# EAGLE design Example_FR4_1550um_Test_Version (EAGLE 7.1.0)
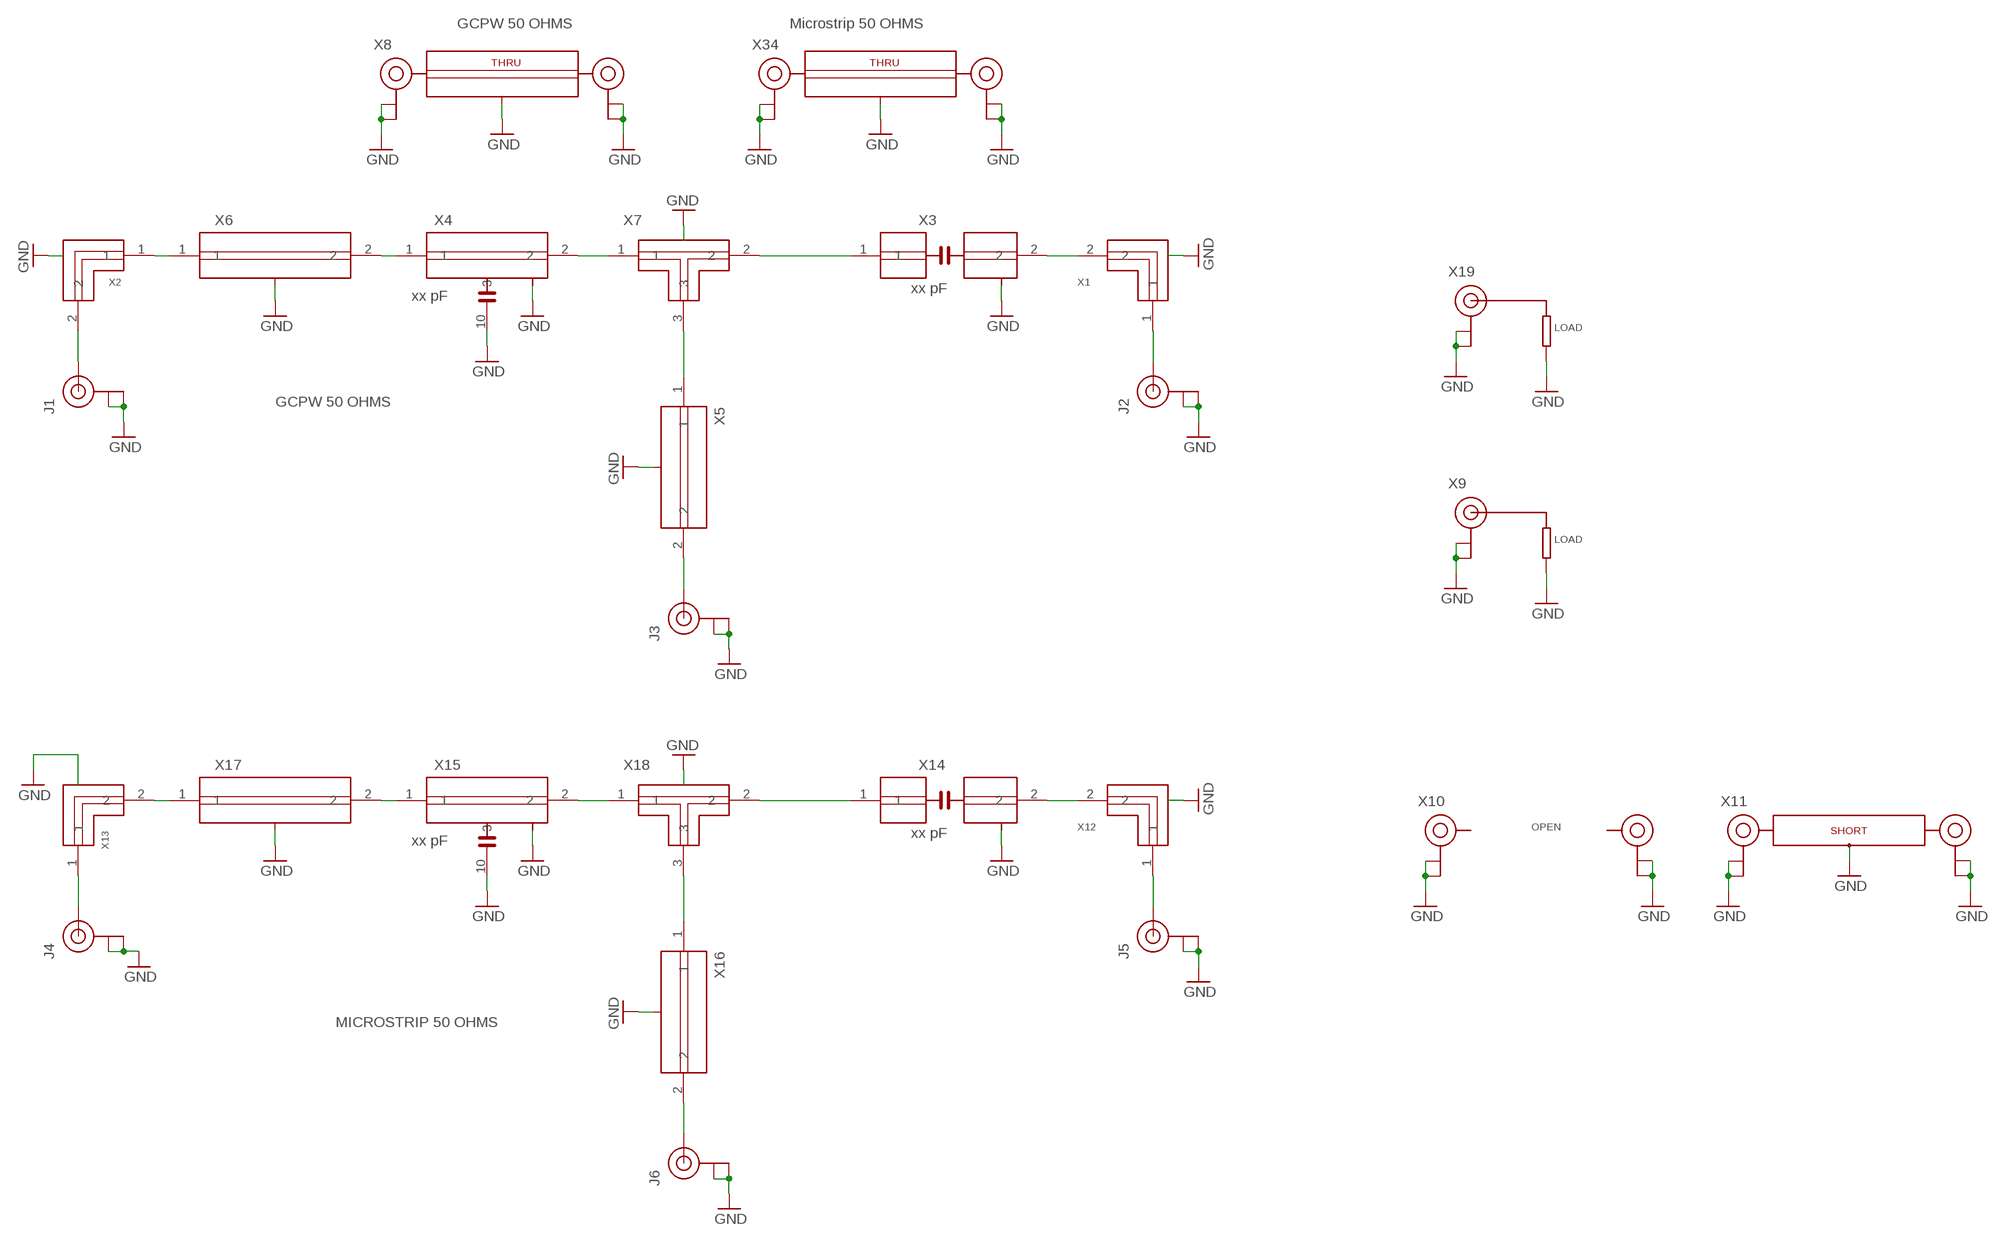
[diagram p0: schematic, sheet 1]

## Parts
J1  U.FL  [U.FL]
J2  U.FL  [U.FL]
J3  U.FL  [U.FL]
J4  U.FL  [U.FL]
J5  U.FL  [U.FL]
J6  U.FL  [U.FL]
X1  CHIPDESIGN_GCPW_50_OHM_L  [GCPW_50_OHM_LEFT]
X2  CHIPDESIGN_GCPW_50_OHM_R  [GCPW_50_OHM_RIGHT]
X3  xx pF  CHIPDESIGN_GCPW_50_OHM_SERIES_0402  [GCPW_50_OHM_0402_SERIES]
X4  xx pF  CHIPDESIGN_GCPW_50_OHM_SHUNT_0402  [GCPW_50_OHM_0402_SHUNT]
X5  CHIPDESIGN_GCPW_50_OHM_TLINE_SHORT  [GCPW_50_OHM_TLINE_SHORT]
X6  CHIPDESIGN_GCPW_50_OHM_TLINE_LONG  [GCPW_50_OHM_TLINE_LONG]
X7  CHIPDESIGN_GCPW_50_OHM_TJUNCTION  [GCPW_50_OHM_TEE]
X8  CHIPDESIGN_GCPW_50_OHM_THRU  [GCPW_50_OHM_THRU]
X9  LOAD_GCPW  [LOAD_GCPW]
X10  OPEN  [OPEN]
X11  SHORT  [SHORT]
X12  CHIPDESIGN_MICROSTRIP_50_OHM_L  [MICROSTRIP_50_OHM_LEFT]
X13  CHIPDESIGN_MICROSTRIP_50_OHM_R  [MICROSTRIP_50_OHM_RIGHT]
X14  xx pF  CHIPDESIGN_MICROSTRIP_50_OHM_SERIES_0402  [MICROSTRIP_50_OHM_0402_SERIES]
X15  xx pF  CHIPDESIGN_MICROSTRIP_50_OHM_SHUNT_0402  [MICROSTRIP_50_OHM_0402_SHUNT]
X16  CHIPDESIGN_MICROSTRIP_50_OHM_TLINE_SHORT  [MICROSTRIP_50_OHM_TLINE_SHORT]
X17  CHIPDESIGN_MICROSTRIP_50_OHM_TLINE_LONG  [MICROSTRIP_50_OHM_TLINE_LONG]
X18  CHIPDESIGN_MICROSTRIP_50_OHM_TJUNCTION  [MICROSTRIP_50_OHM_TEE]
X19  LOAD_MICROSTRIP  [LOAD_MICROSTRIP]
X34  CHIPDESIGN_MICROSTRIP_50_OHM_THRU  [MICROSTRIP_50_OHM_THRU]

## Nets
GND: J1.P$1(GND) J1.P$2(GND) J2.P$1(GND) J2.P$2(GND) J3.P$1(GND) J3.P$2(GND) J4.P$1(GND) J4.P$2(GND) J5.P$1(GND) J5.P$2(GND) J6.P$1(GND) J6.P$2(GND) X1.3(GND) X1.4(GND) X1.5(GND) X1.6(GND) X1.7(GND) X1.8(GND) X1.9(GND) X1.10(GND) X2.3(GND) X2.4(GND) X2.5(GND) X2.6(GND) X2.7(GND) X2.8(GND) X2.9(GND) X2.10(GND) X3.3(GND) X3.4(GND) X3.5(GND) X3.6(GND) X3.7(GND) X3.8(GND) X3.9(GND) X3.10(GND) X3.11(GND) X3.12(GND) X4.3(GND) X4.4(GND) X4.5(GND) X4.6(GND) X4.7(GND) X4.8(GND) X4.9(GND) X4.10 X4.11(GND) X4.12(GND) X5.3(GND) X5.4(GND) X5.5(GND) X5.6(GND) X6.3(GND) X6.4(GND) X6.5(GND) X6.6(GND) X6.7(GND) X6.8(GND) X6.9(GND) X6.10(GND) X6.11(GND) X6.12(GND) X7.4(GND) X7.5(GND) X7.6(GND) X7.7(GND) X7.8(GND) X7.9(GND) X7.10(GND) X7.11(GND) X7.12(GND) X7.13(GND) X7.14(GND) X8.3(GND) X8.4(GND) X8.5(GND) X8.6(GND) X8.7(GND) X8.8(GND) X8.9(GND) X8.10(GND) X8.11(GND) X8.12(GND) X8.P$1(GND) X8.P$2(GND) X8.P$5(GND) X8.P$6(GND) X9.P$1(GND) X9.P$2(GND) X9.P$6(GND) X9.P$7(GND) X9.P$8(GND) X9.P$9(GND) X9.P$10(GND) X9.P$11(GND) X9.P$12(GND) X10.1(GND) X10.2(GND) X10.3(GND) X10.4(GND) X10.5(GND) X10.6(GND) X10.7(GND) X10.8(GND) X10.9(GND) X10.10(GND) X10.11(GND) X10.12(GND) X10.13(GND) X10.14(GND) X10.15(GND) X10.16(GND) X10.17(GND) X10.18(GND) X10.19(GND) X10.20(GND) X10.21(GND) X10.22(GND) X10.23(GND) X10.24(GND) X11.P$1(GND) X11.P$2(GND) X11.P$3(GND) X11.P$5(GND) X11.P$6(GND) X11.P$7(GND) X12.P$1(GND) X12.P$2(GND) X12.P$3(GND) X12.P$4(GND) X12.P$5(GND) X12.P$6(GND) X12.P$7(GND) X12.P$8(GND) X12.P$9(GND) X13.P$1(GND) X13.P$2(GND) X13.P$3(GND) X13.P$4(GND) X13.P$5(GND) X13.P$7(GND) X13.P$8(GND) X13.P$15(GND) X13.P$16(GND) X14.P$1(GND) X14.P$2(GND) X14.P$3(GND) X14.P$4(GND) X14.P$5(GND) X14.P$6(GND) X14.P$7(GND) X14.P$8(GND) X14.P$9(GND) X14.P$10(GND) X15.10 X15.P$1(GND) X15.P$2(GND) X15.P$3(GND) X15.P$4(GND) X15.P$5(GND) X15.P$6(GND) X15.P$7(GND) X15.P$8(GND) X15.P$9(GND) X16.P$1(GND) X16.P$2(GND) X16.P$3(GND) X16.P$4(GND) X17.P$1(GND) X17.P$2(GND) X17.P$3(GND) X17.P$4(GND) X17.P$5(GND) X17.P$6(GND) X17.P$7(GND) X17.P$8(GND) X17.P$9(GND) X17.P$10(GND) X18.P$1(GND) X18.P$2(GND) X18.P$3(GND) X18.P$4(GND) X18.P$5(GND) X18.P$6(GND) X18.P$7(GND) X19.P$1(GND) X19.P$2(GND) X19.P$6(GND) X19.P$7(GND) X19.P$8(GND) X19.P$9(GND) X19.P$10(GND) X19.P$11(GND) X19.P$12(GND) X34.1(GND) X34.2(GND) X34.3(GND) X34.4(GND) X34.5(GND) X34.6(GND) X34.7(GND) X34.8(GND) X34.9(GND) X34.10(GND) X34.11(GND) X34.12(GND) X34.13(GND) X34.14(GND) X34.15(GND) X34.16(GND) X34.17(GND) X34.18(GND) X34.P$1(GND) X34.P$2(GND) X34.P$5(GND) X34.P$6(GND)
N$1: J1.P$3(SIGNAL) X2.2
N$2: X2.1 X6.1
N$3: X4.1 X6.2
N$4: X4.2 X7.1
N$5: X3.1 X7.2
N$6: X5.1 X7.3
N$7: J3.P$3(SIGNAL) X5.2
N$8: X1.2 X3.2
N$9: J2.P$3(SIGNAL) X1.1
N$10: X13.2 X17.1
N$11: J4.P$3(SIGNAL) X13.1
N$13: X15.1 X17.2
N$14: X15.2 X18.1
N$15: X14.1 X18.2
N$16: X16.1 X18.3
N$17: J6.P$3(SIGNAL) X16.2
N$18: X12.2 X14.2
N$19: J5.P$3(SIGNAL) X12.1

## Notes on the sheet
- GCPW 50 OHMS | Microstrip 50 OHMS
- GCPW 50 OHMS
- MICROSTRIP 50 OHMS

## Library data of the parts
J1-J6 = Chipdesign_Isola_050:U.FL: SMD antenna connector- WRL-09144; MPN: U.FL-R-SMT-1(10); OC_NEWARK: 50P8856; PROD_ID: CONN-09193
X1 = Chipdesign_FR4_050:CHIPDESIGN_GCPW_50_OHM_L: Grounded Coplanar Waveguide Line - left; Relative dielectric constant = 4.4; Thickness of dielectric = 1.55mm.; DIELECTRIC: FR4; DK: 4.4; E_EFF: 2.78; OC_NEWARK: unknown; PCB_THICKNESS: 1.55MM; ZO: 50 ohms
X2 = Chipdesign_FR4_050:CHIPDESIGN_GCPW_50_OHM_R: Grounded Coplanar Waveguide Line - right; Relative dielectric constant = 4.4; Thickness of dielectric = 1.55mm.; DIELECTRIC: FR4; DK: 4.4; E_EFF: 2.78; OC_NEWARK: unknown; PCB_THICKNESS: 1.55MM; ZO: 50 ohms
X3 = Chipdesign_FR4_050:CHIPDESIGN_GCPW_50_OHM_SERIES_0402: Grounded Coplanar Waveguide Line - series cap 0402; Relative dielectric constant = 4.4; Thickness of dielectric = 1.55mm.; DIELECTRIC: FR4; DK: 4.4; E_EFF: 2.78; OC_NEWARK: unknown; PCB_THICKNESS: 1.55MM; ZO: 50 ohms
X4 = Chipdesign_FR4_050:CHIPDESIGN_GCPW_50_OHM_SHUNT_0402: Grounded Coplanar Waveguide Line - shunt cap 0402; Relative dielectric constant = 4.4; Thickness of dielectric = 1.55mm.; DIELECTRIC: FR4; DK: 4.4; E_EFF: 2.78; OC_NEWARK: unknown; PCB_THICKNESS: 1.55MM; ZO: 50 ohms
X5 = Chipdesign_FR4_050:CHIPDESIGN_GCPW_50_OHM_TLINE_SHORT: Grounded Coplanar Waveguide Line - TLINE; Relative dielectric constant = 4.4; Thickness of dielectric = 1.55mm.; DIELECTRIC: FR4; DK: 4.4; E_EFF: 2.78; OC_NEWARK: unknown; PCB_THICKNESS: 1.55MM; ZO: 50 Ohms
X6 = Chipdesign_FR4_050:CHIPDESIGN_GCPW_50_OHM_TLINE_LONG: Grounded Coplanar Waveguide Line - TLINE, long; Relative dielectric constant = 4.4; Thickness of dielectric = 1.55mm.; DIELECTRIC: FR4; DK: 4.4; E_EFF: 2.78; OC_NEWARK: unknown; PCB_THICKNESS: 1.55MM; ZO: 50 ohms
X7 = Chipdesign_FR4_050:CHIPDESIGN_GCPW_50_OHM_TJUNCTION: Grounded Coplanar Waveguide - T JUNCTION, long; Relative dielectric constant = 4.4; Thickness of dielectric = 1.55mm.; DIELECTRIC: FR4; DK: 4.4; E_EFF: 2.78; OC_NEWARK: unknown; PCB_THICKNESS: 1.55MM; ZO: 50 ohms
X8 = Chipdesign_FR4_050:CHIPDESIGN_GCPW_50_OHM_THRU: Relative dielectric constant = 4.4; Thickness of dielectric = 1.55mm.; DIELECTRIC: FR4; DK: 4.4; E_EFF: 2.78; OC_NEWARK: unknown; PCB_THICKNESS: 1.55MM; ZO: 50 ohms
X9 = Chipdesign_FR4_050:LOAD_GCPW: Relative dielectric constant = 4.4; Thickness of dielectric = 1.55mm.; OC_NEWARK: unknown
X10 = Chipdesign_FR4_050:OPEN; OC_NEWARK: unknown
X11 = Chipdesign_FR4_050:SHORT: Relative dielectric constant = 4.4; Thickness of dielectric = 1.55mm.; OC_NEWARK: unknown
X12 = Chipdesign_FR4_050:CHIPDESIGN_MICROSTRIP_50_OHM_L: Grounded Coplanar Waveguide Line - left; Relative dielectric constant = 4.4; Thickness of dielectric = 1.55mm.; DIELECTRIC: FR4; DK: 4.4; OC_NEWARK: unknown; PCB_THICKNESS: 1.55MM; TRACK_THICKNESS: 35um; ZO: 50 ohms
X13 = Chipdesign_FR4_050:CHIPDESIGN_MICROSTRIP_50_OHM_R: Grounded Coplanar Waveguide Line - right; Relative dielectric constant = 4.4; Thickness of dielectric = 1.55mm.; DIELECTRIC: FR4; DK: 4.4; OC_NEWARK: unknown; PCB_THICKNESS: 1.55MM; TRACK_THICKNESS: 35um; ZO: 50 ohms
X14 = Chipdesign_FR4_050:CHIPDESIGN_MICROSTRIP_50_OHM_SERIES_0402: Grounded Coplanar Waveguide Line - series cap 0402; Relative dielectric constant = 4.4; Thickness of dielectric = 1.55mm.; DIELECTRIC: FR4; DK: 4.4; OC_NEWARK: unknown; PCB_THICKNESS: 1.55MM; TRACK_THICKNESS: 35um; ZO: 50 ohms
X15 = Chipdesign_FR4_050:CHIPDESIGN_MICROSTRIP_50_OHM_SHUNT_0402: Grounded Coplanar Waveguide Line - shunt cap 0402; Relative dielectric constant = 4.4; Thickness of dielectric = 1.55mm.; DIELECTRIC: FR4; DK: 4.4; OC_NEWARK: unknown; PCB_THICKNESS: 1.55MM; TRACK_THICKNESS: 35um; ZO: 50 ohms
X16 = Chipdesign_FR4_050:CHIPDESIGN_MICROSTRIP_50_OHM_TLINE_SHORT: Grounded Coplanar Waveguide Line - TLINE; Relative dielectric constant = 4.4; Thickness of dielectric = 1.55mm.; DIELECTRIC: FR4; DK: 4.4; OC_NEWARK: unknown; PCB_THICKNESS: 1.55MM; TRACK_THICKNESS: 35um; ZO: 50 ohms
X17 = Chipdesign_FR4_050:CHIPDESIGN_MICROSTRIP_50_OHM_TLINE_LONG: Grounded Coplanar Waveguide Line - TLINE, long; Relative dielectric constant = 4.4; Thickness of dielectric = 1.55mm.; DIELECTRIC: FR4; DK: 4.4; OC_NEWARK: unknown; PCB_THICKNESS: 1.55MM; TRACK_THICKNESS: 35um; ZO: 50 ohms
X18 = Chipdesign_FR4_050:CHIPDESIGN_MICROSTRIP_50_OHM_TJUNCTION: Grounded Coplanar Waveguide - T JUNCTION, long; Relative dielectric constant = 4.4; Thickness of dielectric = 1.55mm.; DIELECTRIC: FR4; DK: 4.4; OC_NEWARK: unknown; PCB_THICKNESS: 1.55MM; TRACK_THICKNESS: 35um; ZO: 50 ohms
X19 = Chipdesign_FR4_050:LOAD_MICROSTRIP: Relative dielectric constant = 4.4; Thickness of dielectric = 1.55mm.; OC_NEWARK: unknown
X34 = Chipdesign_FR4_050:CHIPDESIGN_MICROSTRIP_50_OHM_THRU: Relative dielectric constant = 4.4; Thickness of dielectric = 1.55mm.; DIELECTRIC: FR4; DK: 4.4; OC_NEWARK: unknown; PCB_THICKNESS: 1.55MM; TRACK_THICKNESS: 35um; ZO: 50 ohms

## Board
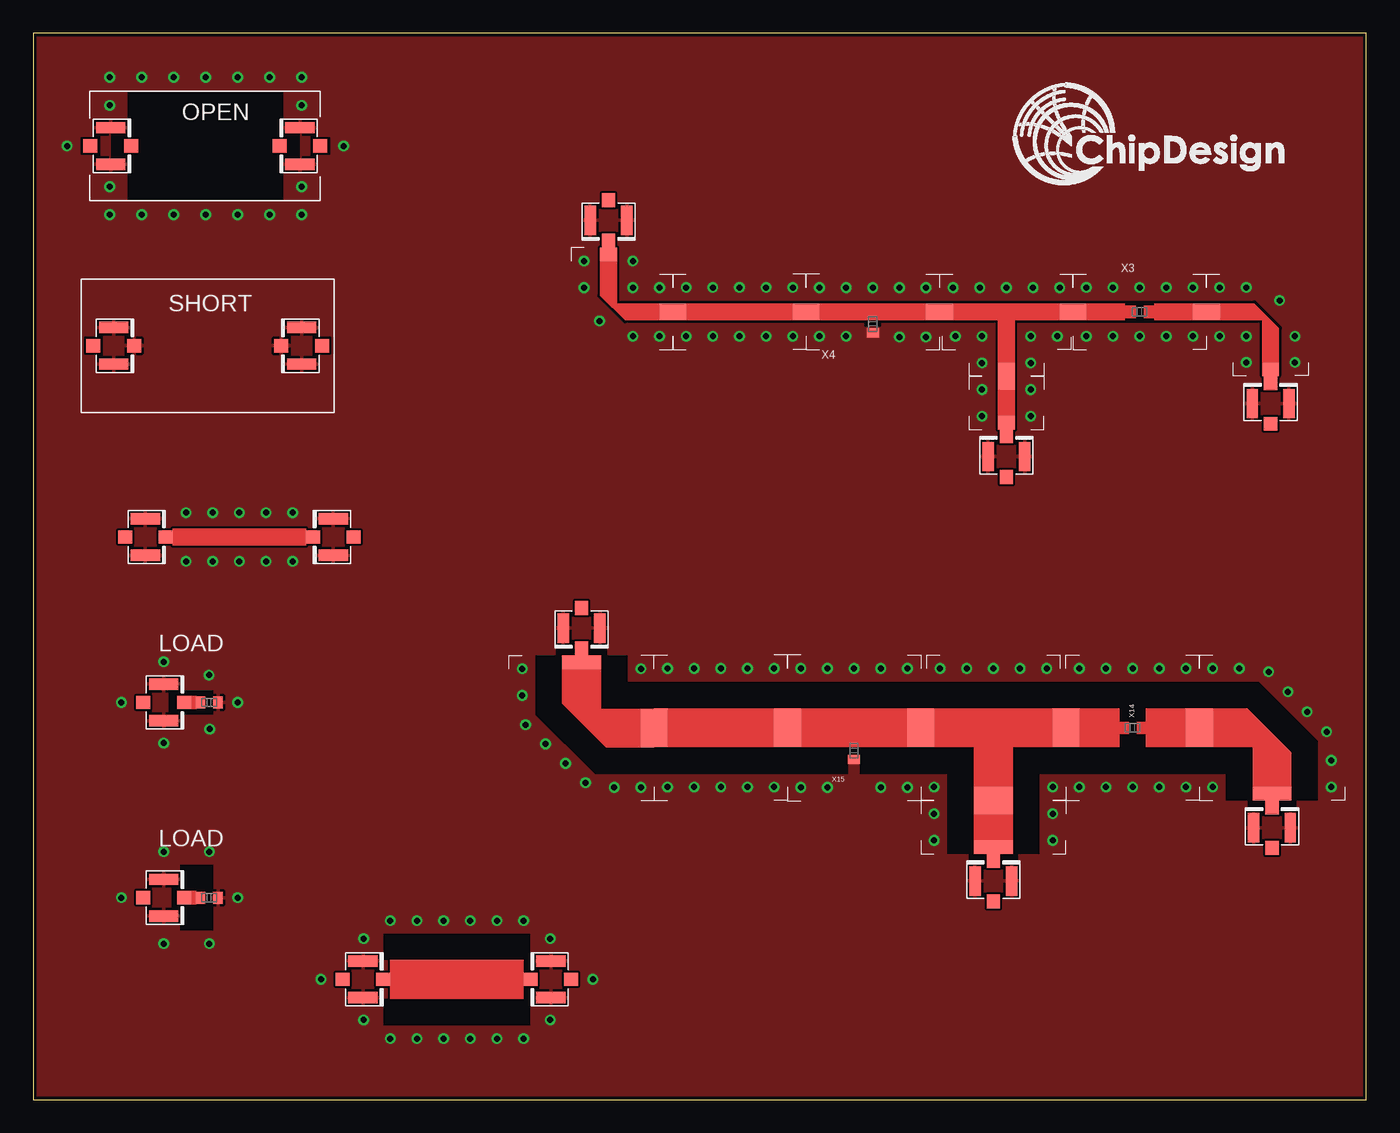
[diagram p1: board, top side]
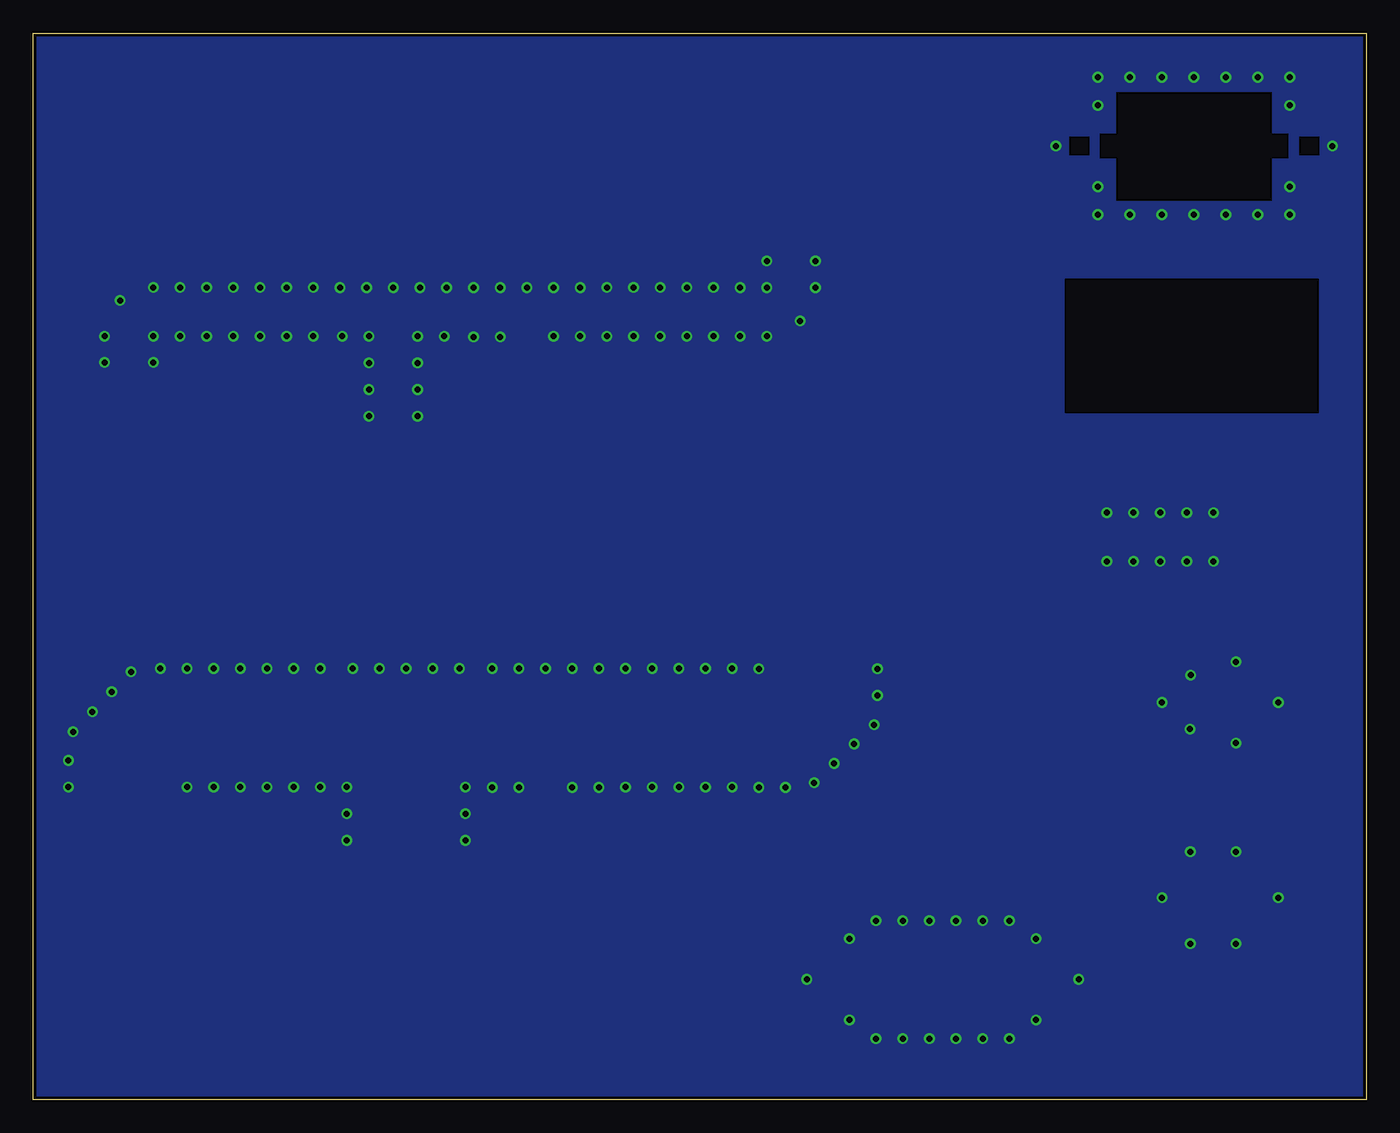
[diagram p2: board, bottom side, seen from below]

Size 100 x 80 mm. Coordinates in mm from the lower left corner, seen from the top.
Outline: 0,0 100,0 100,80 0,80 0,0
Copper layers (1*16): Top 0.035mm / dielectric 1.55mm / Bottom 0.035mm
Design rules "eC_2Layer_PClass6_BaseCopperO35": minimum track width 0.15mm, minimum drill 0.35mm, track to track 0.175mm, track to pad 0.175mm, pad to pad 0.175mm, via to via 0.175mm, smd to smd 0mil, copper to edge 0.25mm, drill to drill 0.35mm, minimum pad ring 0.175mm, minimum via ring 0.125mm, stop-mask expansion 0mil, vias tented up to drill 0.45mm, thermal gap 0.2mm

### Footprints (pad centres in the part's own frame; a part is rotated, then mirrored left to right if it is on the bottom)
U.FL = smd 2.2 x 0.85: P$1 0,1.375; P$2 0,-1.375 | smd 1.05 x 1: P$3 1.525,0; P$4 -1.525,0
GCPW_50_OHM_LEFT = smd 1.25 x 1: 1 4.325,-4.325 | smd 1 x 1.25: 2 0,0 | drill 0.45: 3 2.5,-3.8; 4 2.5,-1.825; 5 0.5,-1.825; 6 0.5,1.825; 7 2.5,1.825; 8 5,0.85; 9 6.15,-1.825; 10 6.15,-3.8
GCPW_50_OHM_RIGHT = smd 1.25 x 1: 1 -4.325,-4.325 | smd 1 x 1.25: 2 0,0 | drill 0.45: 3 -2.5,-3.825; 4 -2.5,-1.825; 5 -0.5,-1.825; 6 -0.5,1.825; 7 -2.5,1.825; 8 -5,0.675; 9 -6.15,-1.825; 10 -6.15,-3.825
GCPW_50_OHM_0402_SERIES = smd 1 x 1.25: 1 -4.5,0; 2 4.5,0 | drill 0.45: 3 -4,1.825; 4 -2,1.825; 5 -4,-1.825; 6 -2,-1.825; 7 2,1.825; 8 2,-1.825; 9 4,-1.825; 10 4,1.825; 11 0,1.825; 12 0,-1.825
GCPW_50_OHM_0402_SHUNT = smd 1 x 1.25: 1 -4.5,0.925; 2 4.5,0.925 | drill 0.45: 3 -4,2.75; 4 -2,2.75; 5 0,2.75; 6 2,2.75; 7 4,2.75; 8 -4,-0.9; 9 -2,-0.9; 11 2,-0.95; 12 4,-0.95 | smd 0.9 x 0.7: 10 0,-0.65
GCPW_50_OHM_TLINE_SHORT = smd 1 x 1.25: 1 0,0; 2 3,0 | drill 0.45: 3 0.5,1.825; 4 2.5,1.825; 5 0.5,-1.825; 6 2.5,-1.825
GCPW_50_OHM_TLINE_LONG = smd 1 x 1.25: 1 0,0; 2 9,0 | drill 0.45: 3 0.5,1.825; 4 2.5,1.825; 5 0.5,-1.825; 6 2.5,-1.825; 7 4.5,1.825; 8 4.5,-1.825; 9 6.5,-1.825; 10 6.5,1.825; 11 8.5,1.825; 12 8.5,-1.825
GCPW_50_OHM_TEE = smd 1 x 1.25: 1 -4.5,4.325; 2 4.5,4.325 | smd 1.25 x 1: 3 0,0 | drill 0.45: 4 -3.825,2.5; 5 -1.825,2.5; 6 -1.825,0.5; 7 1.825,0.5; 8 1.825,2.5; 9 3.825,2.5; 10 4,6.15; 11 2,6.15; 12 0,6.15; 13 -2,6.15; 14 -4,6.15
GCPW_50_OHM_THRU = drill 0.45: 3 0.5,1.825; 4 2.5,1.825; 5 0.5,-1.825; 6 2.5,-1.825; 7 4.5,1.825; 8 4.5,-1.825; 9 6.5,-1.825; 10 6.5,1.825; 11 8.5,1.825; 12 8.5,-1.825 | smd 2.2 x 0.85: P$1 -2.55,1.375; P$2 -2.55,-1.375; P$5 11.55,-1.375; P$6 11.55,1.375 | smd 1.05 x 1: P$3 -1.025,0; P$4 -4.075,0; P$7 10.025,0; P$8 13.075,0
LOAD_GCPW = smd 2.2 x 0.85: P$1 -3.425,1.375; P$2 -3.425,-1.375 | smd 1.05 x 1: P$3 -1.9,0; P$4 -4.95,0 | smd 0.7 x 0.9: P$5 -0.65,0; P$6 0.65,0 | drill 0.45: P$7 2.125,0; P$8 -0.025,2.05; P$9 -3.425,3.05; P$10 -6.6,0; P$11 -3.425,-3.05; P$12 0.025,-2
OPEN = drill 0.45: 1 -1.6,-3.05; 4 -1.6,3.05; 5 12.8,3.05; 8 12.8,-3.05; 9 -1.6,-5.15; 10 0.8,-5.15; 11 3.2,-5.15; 12 5.6,-5.15; 13 8,-5.15; 14 10.4,-5.15; 15 12.8,-5.15; 16 -1.6,5.15; 17 0.8,5.15; 18 3.2,5.15; 19 5.6,5.15; 20 8,5.15; 21 10.4,5.15; 22 12.8,5.15; 23 -4.8,0; 24 15.95,0 | smd 2.2 x 0.85: 2 -1.525,-1.375; 3 -1.525,1.375; 6 12.675,1.375; 7 12.675,-1.375 | smd 1.05 x 1: P$3 0,0; P$4 -3.05,0; P$7 11.15,0; P$8 14.2,0
SHORT = smd 2.2 x 0.85: P$1 -1.55,1.375; P$2 -1.55,-1.375; P$5 12.55,-1.375; P$6 12.55,1.375 | smd 1.05 x 1: P$3 -0.025,0; P$4 -3.075,0; P$7 11.025,0; P$8 14.075,0
MICROSTRIP_50_OHM_LEFT = smd 2.9 x 1: 1 4.95,-4.95 | smd 1 x 2.9: 2 0,0 | drill 0.45: P$1 0.5,4.45; P$2 2.5,4.45; P$3 0.5,-4.45; P$4 9.4,-4.45; P$5 9.4,-2.45; P$6 4.7,4.2; P$7 7.6,1.2; P$8 6.15,2.7; P$9 9.05,-0.3
MICROSTRIP_50_OHM_RIGHT = smd 1 x 2.9: 1 0,0 | smd 2.9 x 1: 2 -4.95,-4.95 | drill 0.45: P$1 -9.4,-4.45; P$2 -9.4,-2.45; P$3 -0.5,-4.45; P$4 -0.5,4.45; P$5 -2.5,4.45; P$7 -6.15,2.7; P$8 -7.6,1.2; P$15 -4.7,4.2; P$16 -9.05,-0.3
MICROSTRIP_50_OHM_0402_SERIES = smd 1 x 2.9: 1 -4.5,0; 2 4.5,0 | drill 0.45: P$1 -4,4.45; P$2 -2,4.45; P$3 0,4.45; P$4 2,4.45; P$5 4,4.45; P$6 -4,-4.45; P$7 -2,-4.45; P$8 0,-4.45; P$9 2,-4.45; P$10 4,-4.45
MICROSTRIP_50_OHM_0402_SHUNT = smd 1 x 2.9: 1 -4.5,1.725; 2 4.5,1.725 | smd 0.9 x 0.7: 10 0,-0.65 | drill 0.45: P$1 -4,6.175; P$2 -2,6.175; P$3 0,6.175; P$4 2,6.175; P$5 4,6.175; P$6 -4,-2.75; P$7 -2,-2.75; P$8 4,-2.75; P$9 2,-2.75
MICROSTRIP_50_OHM_TLINE_SHORT = smd 1 x 2.9: 1 0,0; 2 3,0 | drill 0.45: P$1 0.5,4.45; P$2 2.5,4.45; P$3 0.5,-4.45; P$4 2.5,-4.45
MICROSTRIP_50_OHM_TLINE_LONG = smd 1 x 2.9: 1 0,0; 2 9,0 | drill 0.45: P$1 0.5,4.45; P$2 8.5,4.45; P$3 0.5,-4.45; P$4 8.5,-4.45; P$5 2.5,4.45; P$6 4.5,4.45; P$7 6.5,4.45; P$8 2.5,-4.45; P$9 4.5,-4.45; P$10 6.5,-4.45
MICROSTRIP_50_OHM_TEE = smd 1 x 2.9: 1 -4.95,4.95; 2 4.95,4.95 | smd 2.9 x 1: 3 0,0 | drill 0.45: P$1 -4,9.4; P$2 4,9.4; P$3 -2,9.4; P$4 0,9.4; P$5 -4.45,0.5; P$6 2,9.4; P$7 4.45,0.5
LOAD_MICROSTRIP = smd 2.2 x 0.85: P$1 -3.425,1.375; P$2 -3.425,-1.375 | smd 1.05 x 1: P$3 -1.9,0; P$4 -4.95,0 | smd 0.7 x 0.9: P$5 -0.65,0; P$6 0.65,0 | drill 0.45: P$7 2.125,0; P$8 0,3.45; P$9 -3.425,3.45; P$10 -6.6,0; P$11 -3.425,-3.45; P$12 0,-3.45
MICROSTRIP_50_OHM_THRU = drill 0.45: 1 -0.5,4.4; 2 1.5,4.4; 3 -2.5,3.05; 4 -5.7,0; 5 -2.5,-3.05; 6 11.5,-3.05; 7 14.7,0; 8 11.5,3.05; 9 3.5,4.4; 10 5.5,4.4; 11 7.5,4.4; 12 9.5,4.4; 13 -0.5,-4.45; 14 1.5,-4.45; 15 3.5,-4.45; 16 5.5,-4.45; 17 7.5,-4.45; 18 9.5,-4.45 | smd 2.2 x 0.85: P$1 -2.55,1.375; P$2 -2.55,-1.375; P$5 11.55,-1.375; P$6 11.55,1.375 | smd 1.05 x 1: P$3 -1.025,0; P$4 -4.075,0; P$7 10.025,0; P$8 13.075,0

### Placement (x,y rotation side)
J1  43.15,65.97 270 top
J2  92.83,52.23 90 top
J3  73,48.25 90 top
J4  41.12,35.38 270 top
J5  92.92,20.4 90 top
J6  72.03,16.4 90 top
X1  88.5,59.1 0 top
X2  43.15,63.42 90 top
X3  83,59.1 0 top
X4  62.98,58.17 0 top
X5  73,53.77 270 top
X6  48.48,59.1 0 top
X7  73,54.77 0 top
X8  10.96,42.21 0 top
X9  13.2,29.79 0 top
X10  7.33,71.55 0 top
X11  7.58,56.56 0 top
X12  87.97,27.9 0 top
X13  41.12,32.83 90 top
X14  82.47,27.9 0 top
X15  61.58,26.18 0 top
X16  72.03,21.95 270 top
X17  47.08,27.9 0 top
X18  72.03,22.95 0 top
X19  13.2,15.15 0 top
X34  27.27,9.03 0 top

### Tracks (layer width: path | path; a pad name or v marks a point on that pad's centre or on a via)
GND
  pour Top: 0,0 100,0 100,80 0,80
  pour Bottom: 0,0 100,0 100,80 0,80
N$1
  Top 0.15: J1.P$3 43.16,64.3 43.16,63.49 X2.2
N$2
  Top 0.15: X2.1 47.61,59.15 48.42,59.15 X6.1
N$3
  Top 0.15: X6.2 57.52,59.15 58.34,59.15 X4.1
N$4
  Top 0.15: X4.2 67.6,59.15 68.41,59.15 X7.1
N$5
  Top 0.15: X7.2 77.51,59.15 78.49,59.15 X3.1
N$6
  Top 0.15: X5.1 73.12,53.79 73.12,54.76 X7.3
N$7
  Top 0.15: J3.P$3 73.12,49.89 73.12,50.7 X5.2
N$8
  Top 0.15: X3.2 87.59,59.15 88.4,59.15 X1.2
N$9
  Top 0.15: J2.P$3 92.95,53.79 92.95,54.76 X1.1
N$10
  Top 0.15: X13.2 46.15,27.95 46.96,27.95 X17.1
N$11
  Top 0.15: J4.P$3 41.27,33.8 41.27,32.83 X13.1
N$12
  cutout Top: 39.2,33.4 40.45,33.4 40.45,34.15 39.2,34.15
  cutout Top: 41.8,33.4 43.05,33.4 43.05,34.15 41.8,34.15
  cutout Top: 70.2,17.6 71.45,17.6 71.45,18.35 70.2,18.35
  cutout Top: 72.6,17.6 73.85,17.6 73.85,18.35 72.6,18.35
N$13
  Top 0.15: X17.2 56.23,27.95 57.04,27.95 X15.1
N$14
  Top 0.15: X15.2 66.14,27.95 66.95,27.95 X18.1
N$15
  Top 0.15: X18.2 77.03,27.95 77.84,27.95 X14.1
N$16
  Top 0.15: X16.1 72.15,22.1 72.15,22.91 X18.3
N$17
  Top 0.15: J6.P$3 72.15,18.04 72.15,18.85 X16.2
N$18
  Top 0.15: X14.2 87.1,27.95 87.91,27.95 X12.2
N$19
  Top 0.15: J5.P$3 92.95,21.94 92.95,22.91 X12.1
N$20
  cutout Top: 93.5,21.6 94.75,21.6 94.75,22.35 93.5,22.35
  cutout Top: 91.1,21.6 92.35,21.6 92.35,22.35 91.1,22.35
N$21
  cutout Top: 36.9,11.05 37.65,11.05 37.65,9.7 36.9,9.7
  cutout Top: 37.65,7.1 36.9,7.1 36.9,8.45 37.65,8.45

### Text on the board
tDocu: GCPW 50 OHM | MICROSTRIP 50 OHM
